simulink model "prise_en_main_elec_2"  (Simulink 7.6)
settings: Solver=ode15s  StartTime=0.0  StopTime=10  RelTol=1e-3
InitFcn:
  | R=1e3;    % 1 Kohm
  | C=1e-3;  % 1 mF
  | U0=5       % échelon d'entrée en V
  | 
  | clc
  | delete *.mat
StopFcn:
  | load appli_circuit_RC.mat
  | plotyy(x(1,:),x(3,:),x(1,:),x(4,:))
  | title('Tension aux bornes de C et courant dans le circuit RC')
  | grid
  | axis([0 10 -0.5 5.5])
  | xlabel('temps')
libraries: fl_lib x9, nesl_utility x5, elec_lib x1

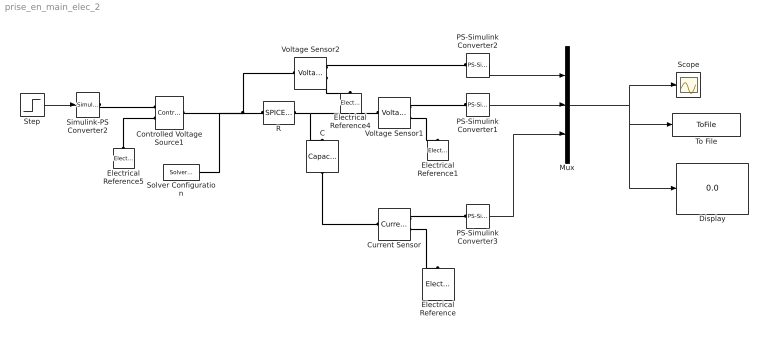
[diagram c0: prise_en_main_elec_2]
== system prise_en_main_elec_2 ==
  C : fl_lib/Electrical/Electrical Elements/Capacitor  DialogController=NetworkEngine.DynNeDlgSource  SystemSampleTime=-1  c=C F  v0=0 V  r=1e-06 Ohm  g=0 1/Ohm  i_Log=off  v_Log=off  vc_Log=off  LocalVarNames=|i|v|vc  LocalVarDescs=|i|v|Internal variable for voltage across capacitor term  LocalVarLogging=[0 0 0]
  Controlled Voltage Source1 : fl_lib/Electrical/Electrical Sources/Controlled Voltage Source  DialogController=NetworkEngine.DynNeDlgSource  SystemSampleTime=-1  i_Log=off  v_Log=off  LocalVarNames=|current|voltage|power  LocalVarDescs=|Current (A)|Voltage (V)|Power (W)  LocalVarLogging=[0 0 0]
  Current Sensor : fl_lib/Electrical/Electrical Sensors/Current Sensor  DialogController=NetworkEngine.DynNeDlgSource  SystemSampleTime=-1  i1_Log=off  v1_Log=off  LocalVarNames=|i1|v1  LocalVarDescs=|i1|v1  LocalVarLogging=[0 0]
  Display : Display
  Electrical Reference : fl_lib/Electrical/Electrical Elements/Electrical Reference  DialogController=NetworkEngine.DynNeDlgSource  SystemSampleTime=-1  i_Log=off  LocalVarNames=|i  LocalVarDescs=|i  LocalVarLogging=0
  Electrical Reference1 : fl_lib/Electrical/Electrical Elements/Electrical Reference  DialogController=NetworkEngine.DynNeDlgSource  SystemSampleTime=-1  i_Log=off  LocalVarNames=|i  LocalVarDescs=|i  LocalVarLogging=[]
  Electrical Reference4 : fl_lib/Electrical/Electrical Elements/Electrical Reference  DialogController=NetworkEngine.DynNeDlgSource  SystemSampleTime=-1  i_Log=off  LocalVarNames=|i  LocalVarDescs=|i  LocalVarLogging=[]
  Electrical Reference5 : fl_lib/Electrical/Electrical Elements/Electrical Reference  DialogController=NetworkEngine.DynNeDlgSource  SystemSampleTime=-1  i_Log=off  LocalVarNames=|i  LocalVarDescs=|i  LocalVarLogging=[]
  Mux : Mux  Inputs=3
  PS-Simulink Converter1 : nesl_utility/PS-Simulink Converter  DialogController=NetworkEngine.DynNeUtilDlgSource  SystemSampleTime=-1  PhysicalDomain=network_engine_domain  LeftPortType=input  RightPortType=output  SubClassName=ps_output  Unit=1  AffineConversion=off
  PS-Simulink Converter2 : nesl_utility/PS-Simulink Converter  DialogController=NetworkEngine.DynNeUtilDlgSource  SystemSampleTime=-1  PhysicalDomain=network_engine_domain  LeftPortType=input  RightPortType=output  SubClassName=ps_output  Unit=1  AffineConversion=off
  PS-Simulink Converter3 : nesl_utility/PS-Simulink Converter  DialogController=NetworkEngine.DynNeUtilDlgSource  SystemSampleTime=-1  PhysicalDomain=network_engine_domain  LeftPortType=input  RightPortType=output  SubClassName=ps_output  Unit=A  AffineConversion=off
  R : elec_lib/Additional Components/SPICE-Compatible Components/Passive Devices/SPICE Resistor  DialogController=NetworkEngine.DynNeDlgSource  SystemSampleTime=-1  SCALE=1  R_param=1  R=R Ohm  RSH=0 Ohm  LENGTH=1e-06 m  WIDTH=1e-06 m  NARROW=0 m  T_param=1  TC1=0 1/K  TC2=0 1/K^2  TOFFSET=0 K  TFIXED=300.15 K  TMEAS=300.15 K  LocalVarLogging=[]
  Scope : Scope
  Simulink-PS Converter2 : nesl_utility/Simulink-PS Converter  DialogController=NetworkEngine.DynNeUtilDlgSource  SystemSampleTime=-1  PhysicalDomain=network_engine_domain  LeftPortType=input  RightPortType=output  SubClassName=ps_input  Unit=1  AffineConversion=off  InputFilterTimeConstant=.001  UdotUserProvided=0
  Solver Configuration : nesl_utility/Solver Configuration  DialogController=NetworkEngine.DynNeUtilDlgSource  SystemSampleTime=-1  PhysicalDomain=network_engine_domain  LeftPortType=input  RightPortType=generic  SubClassName=solver  Accelerate=off  Profile=off  ResidualTolerance=1e-9  MaxNonlinIter=12  MaxModeIter=2  DoFixedCost=off  UseLocalSampling=off  DoDC=off  LinearAlgebra=Sparse  LocalSolverSampleTime=.001  LocalSolverChoice=NE_BACKWARD_EULER_ADVANCER  UseLocalSolver=off
  Step : Step  After=U0  SampleTime=0
  To File : ToFile  Filename=appli_circuit_RC  MatrixName=x
  Voltage Sensor1 : fl_lib/Electrical/Electrical Sensors/Voltage Sensor  DialogController=NetworkEngine.DynNeDlgSource  SystemSampleTime=-1  i1_Log=off  v1_Log=off  LocalVarNames=|i1|v1  LocalVarDescs=|i1|v1  LocalVarLogging=[]
  Voltage Sensor2 : fl_lib/Electrical/Electrical Sensors/Voltage Sensor  DialogController=NetworkEngine.DynNeDlgSource  SystemSampleTime=-1  i1_Log=off  v1_Log=off  LocalVarNames=|i1|v1  LocalVarDescs=|i1|v1  LocalVarLogging=[]
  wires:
  PS-Simulink Converter2/1 -> Mux/1
  Step/1 -> Simulink-PS Converter2/1
  PS-Simulink Converter1/1 -> Mux/2
  Mux/1 -> Scope/1, To File/1, Display/1
  PS-Simulink Converter3/1 -> Mux/3
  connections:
  R/RConn1 -- C/LConn1 -- Voltage Sensor1/LConn1
  Voltage Sensor2/RConn1 -- PS-Simulink Converter2/LConn1
  Electrical Reference5/LConn1 -- Controlled Voltage Source1/RConn2
  Simulink-PS Converter2/RConn1 -- Controlled Voltage Source1/RConn1
  Voltage Sensor2/LConn1 -- R/LConn1 -- Controlled Voltage Source1/LConn1 -- Solver Configuration/RConn1
  Voltage Sensor1/RConn1 -- PS-Simulink Converter1/LConn1
  Voltage Sensor1/RConn2 -- Electrical Reference1/LConn1
  Voltage Sensor2/RConn2 -- Electrical Reference4/LConn1
  C/RConn1 -- Current Sensor/LConn1
  Current Sensor/RConn2 -- Electrical Reference/LConn1
  Current Sensor/RConn1 -- PS-Simulink Converter3/LConn1
